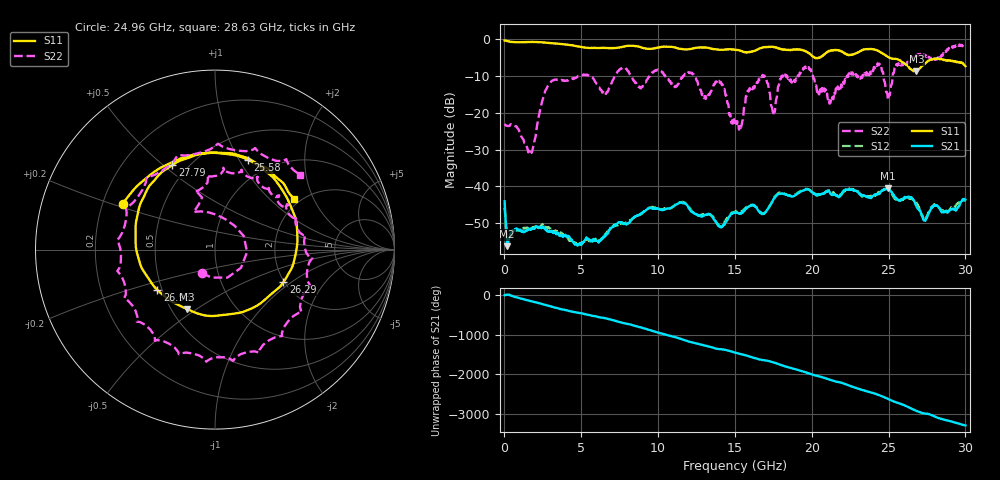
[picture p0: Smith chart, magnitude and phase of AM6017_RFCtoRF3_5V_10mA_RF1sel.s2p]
!Agilent Technologies,E8364B,MY43040894,A.07.50.67
!Agilent E8364B: A.07.50.67
!Date: Tuesday, August 21, 2018 13:40:14
!Correction: S11(Full 2 Port(1,2))
!S21(Full 2 Port(1,2))
!S12(Full 2 Port(1,2))
!S22(Full 2 Port(1,2))
!S2P File: Measurements: S11, S21, S12, S22:
# Hz S  dB  R 50
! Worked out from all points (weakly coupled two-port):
!   1601 points, 10 MHz to 30 GHz, reference 50 ohm
!   highest |S21| = -40.52 dB at 24.94 GHz (marker M1); lowest = -56.2 dB at 178.7 MHz (marker M2)
!   lowest |S11| = -8.7 dB at 26.81 GHz (marker M3), VSWR 2.15, Z = 29.9 - j22.8 ohm
!   |S11| at or under -10 dB: nowhere
!   |S22| runs from -31.1 to -1.2 dB; largest |S21 - S12| = 0.011
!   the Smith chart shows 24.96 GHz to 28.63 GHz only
!   S11 on the Smith chart (normalised r, x): 24.96 GHz: 0.29, +0.22; 25.58 GHz: 0.78, +1.09; 26.29 GHz: 1.98, -0.87; 26.98 GHz: 0.47, -0.25; 27.79 GHz: 0.41, +0.54; 28.63 GHz: 1.87, +1.44
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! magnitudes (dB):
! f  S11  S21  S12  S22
! 10 MHz  -0.4  -44.0  -45.8  -23.0
! 178.7 MHz  -0.5  -56.2  -54.2  -23.6
! 1.678 GHz  -0.8  -51.7  -51.4  -31.1
! 2.897 GHz  -1.1  -52.2  -51.2  -12.2
! 5.015 GHz  -2.2  -55.8  -55.2  -9.7
! 10.02 GHz  -2.3  -46.1  -45.9  -8.5
! 13.97 GHz  -2.9  -50.8  -50.8  -11.3
! 15.01 GHz  -2.9  -47.1  -46.8  -23.4
! 16.69 GHz  -2.5  -47.2  -47.0  -10.1
! 17.5 GHz  -2.1  -43.5  -43.3  -20.4
! 20.01 GHz  -4.6  -41.6  -41.5  -9.2
! 24.3 GHz  -3.2  -42.1  -41.9  -6.7
! 24.94 GHz  -4.8  -40.5  -40.5  -15.8
! 24.96 GHz  -4.8  -40.6  -40.6  -16.5
! 25.01 GHz  -5.0  -40.8  -40.7  -15.0
! 25.58 GHz  -5.5  -43.5  -43.6  -7.2
! 26.29 GHz  -7.5  -42.8  -43.1  -6.5
! 26.81 GHz  -8.7  -45.5  -44.3  -4.3
! 26.98 GHz  -8.1  -46.4  -45.6  -4.5
! 27.79 GHz  -5.6  -46.0  -45.6  -5.5
! 28.63 GHz  -5.6  -46.9  -46.9  -4.0
! 30 GHz  -7.4  -43.6  -43.8  -1.2
